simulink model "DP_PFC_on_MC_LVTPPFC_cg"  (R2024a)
settings: Solver=FixedStepDiscrete  StartTime=0.0  StopTime=0.2  FixedStep=10e-6  RelTol=1e-3  EnableMultiTasking=on
model workspace (MAT data in the model file):
  Freq = 100
  Phas = 0
  SinFreq_1 = 250
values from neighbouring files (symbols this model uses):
  ADC = ADCType.Noise    [TotemPole_PFCData.m]
  Control = ControlType.Simple    [TotemPole_PFCData.m]
  Tsc_slow = 0.01    [TotemPole_PFCData.m]
undefined symbols (not defined in the file or in its folder): a, A0, A8, AD1, AD2, AD3, AD4, AD5, address, also, AN11, AN2, AN3, AN5, AN6, AppData, as, B0, B10, B11, B7, B8, below, bin2dec, bit, bits, BOR, C, C6, C7, C9, cause, characters, Code, Communicate, contains, counter, D, D4, Data, data, dead, default, Detailed, deviced, disasserted, DS70005539, dsPIC33AK128MC106, EC, ECIO, ensure, events, Family, faster, Floating, fulll, highest, HS, HS3, I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
libraries: MCHP_Blockset x16, simulink x4, dspswit3 x1
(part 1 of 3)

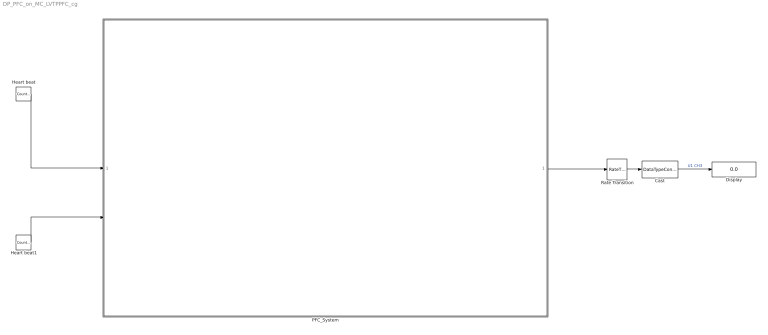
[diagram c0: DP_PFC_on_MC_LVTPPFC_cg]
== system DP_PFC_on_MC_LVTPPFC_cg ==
  Cast : DataTypeConversion  OutDataTypeStr=single
  Display : Display
  Heart beat : simulink/Sources/Counter Free-Running  NumBits=1  tsamp=.25
  Heart beat1 : simulink/Sources/Counter Free-Running  NumBits=1  tsamp=.125
  PFC_System : Subsystem
  Rate Transition : RateTransition  OutPortSampleTime=1
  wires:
  Heart beat/1 -> PFC_System/1(LED2 PIM)
  Heart beat1/1 -> PFC_System/2(LED0 Board)
  PFC_System/1(MCU load) -> Rate Transition/1
  Cast/1 -> Display/1  "U1 CH3"
  Rate Transition/1 -> Cast/1

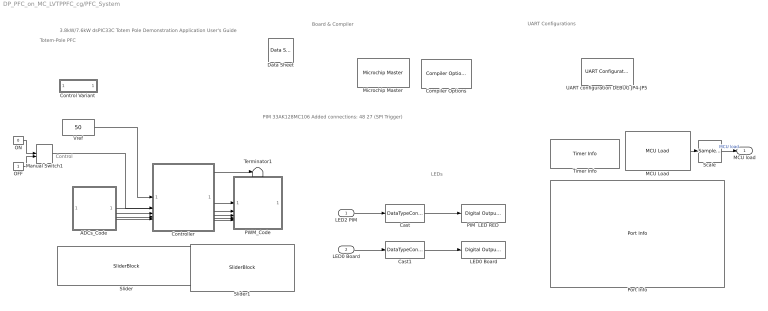
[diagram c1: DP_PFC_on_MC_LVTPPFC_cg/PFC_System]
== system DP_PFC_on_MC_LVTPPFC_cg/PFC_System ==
  note: 3.8kW/7.6kW dsPIC33C Totem Pole Demonstration Application User's Guide
  note: PIM 33AK128MC106 Added connections: 48 27 (SPI Trigger)
  note: UART Configurations
  note: LEDs
  note: Board & Compiler
  note: Control
  note: Totem-Pole PFC
  LED2 PIM : Inport
  LED0 Board : Inport  Port=2
  " LED0 Board" : MCHP_Blockset/Digital IO/Digital Output Write  PORT=Dynamic Options  PORT_TXT="C   [ 0 : 11 ]"  PIN=11  INIT_VALUE=-1  PACK=off  OUTPUT_PIN_MODE=Push-Pull (default)  SIMULTANEOUS=off  ORDERING=None  SampleTime=-1  MCHP_PORT={Digital Out}{DOU}1:1:C11;  MCHP_MASTERLINK=TotemPole_PFC_CodeGen/PFC_System/Control Variant /Microchip Master1
  ADCs_Code : Subsystem  VariantControl=ADC == 3
  Cast : DataTypeConversion  OutDataTypeStr=boolean
  Cast1 : DataTypeConversion  OutDataTypeStr=boolean
  Compiler Options : MCHP_Blockset/System Configuration/Compiler Options  Priority=1  LATEST_CMPLR=off  COMP_LIST=Dynamic Options  COMP_LIST_TXT=XC-DSC - v3.19  DFP_LIST=Dynamic Options  DFP_LIST_TXT=v 1.0.33  CMSIS_DSP=Dynamic Options  CMSIS_DSP_TXT=Dynamic Options  USE_64BIT_DOUBLE=on  MCHP_MULTITHREAD_COMPILATION=on  UseCustom_LinkerScript=off  MCHP_MASTERLINK=TotemPole_PFC_CodeGen/PFC_System/Control Variant /Microchip Master1  OPTIMIZATION_LEVEL=3  MPLAB_LINKLIB=default  MPLAB_LINKLIB1=default  CodeReplacement=Dynamic Options  CodeReplacement_TXT=None  OPTIMIZATION_FLTO=on  OPTIMIZATION_REORDER=off  OPTIMIZATION_ASM_REORDER=on  UNROLL_LOOPS=off  PROCEDURAL_ABSTRACTION=off  CONSERVE_STACK=off  GC_SECTIONS=None  MCODE=is less than 32768 (faster)  MCONST=in code memory  MDATA=Can use all available memory  MSCALAR=Use only memory below address 8192 (faster)  MLARGEARRAY=off  MAGGREGATE=on  HEAP_SIZE=0  OMF=elf  DEBUG_INFO=on  MCHP_STACK_USAGE=off  GCC_STACK_USAGE=off  ProduceHexOutput=off  AssemblyListing=off  SaveTemps=off  NO_EDS_WARN=on  PRINT_STATISTICS=off
  "Control Variant " : Subsystem  mask(Variant Selections){ControlVar=Detailed, IControlVar=PI}
      mask prompts: ControlVar "Control Variant"; IControlVar "IControl Variant"
      mask help: Select the configuration variants here.
  Controller : Subsystem  TreatAsAtomicUnit=on  ReferencedSubsystem=Control
  Data Sheet : MCHP_Blockset/System Info/Data Sheet  DOC_Type=datasheet  DOC_MCHP_Id=33AK128MC106_datasheet  DOC_FilePath=C:\Users\m67135\AppData\Local\Temp\dsPIC33AK128MC106-Family-Data-Sheet-DS70005539.pdf  DOC_FileLastCheckTime="[2024             11             14             11             58         37.374]"  cpy_MCHP_Id=33AK128MC106  MCHP_MASTERLINK=TotemPole_PFC_CodeGen/PFC_System/Control Variant /Microchip Master1
  MCU Load : MCHP_Blockset/Profiling/MCU Load  MCULoadPin=Dynamic Options  MCULoadPin_TXT=None  MCULoadMeasure=on  TIMER_Resolution=Dynamic Options  TIMER_Resolution_TXT="Resol: 0.005(us)  -  Max: 0.328(ms)"  MCHP_TIMER_REQUEST={MCU_Load}{MCU_Load}21:5:0:0:[]:32768;  MCHP_TIMER_RESULT=[2 65535 ]  MCHP_MASTERLINK=TotemPole_PFC_CodeGen/PFC_System/Control Variant /Microchip Master1  MCHP_COMPILED_INFO="CompiledSampleTime= [0.00020000000000000000958   0 ];CompiledInportDataTypes=[    ];CompiledInportDataWidth=[];"  Info="Timer 2:  Resol: 5(ns)  -  Max: 327.68(us)"  SampleTime=.0002
  Manual Switch1 : ManualSwitch  CurrentSetting=0
  Microchip Master : MCHP_Blockset/System Configuration/Microchip Master  Priority=1  PICREF=33AK128MC106  TIMESTEP_REF=PWM1_Trg1 + ADC  BUSYFLAG=Dynamic Options  BUSYFLAG_TXT=B10 / Pin[31]  VDD_range=Dynamic Options  PWRTEN=Not used  BOREN=Disable  BODENV=2.7V  BORV=Not used  FPWRT=128ms  DSBOREN=Enable ZPBOR during Deep Sleep Mode  DSLPBOR=Not used  MCLRE=Enabled  SMCLR=MCLR pin generates a normal system Reset  PMDL1WAY=Allow only one reconfiguration  RSTPRI=Device will obtain reset instruction from Primary flash  TEMP=Not used  SOSCSRC=Not used  SOSCSEL=Not used  IOL1WAY=Allow only one reconfiguration  ALTVREF=Not used  DISUVREG=Not used  DSSWEN=Not used  LPCFG=Not used  RTCBAT=Not used  VBTBOR=Not used  WUTSEL=Not used  POWERSAVE=off  FNOSC=Primary Oscillator (XT; HS; EC)  FPR=ECIO w/ PLL 16x  FOSFPR=HS3 w/PLL 16x  FOS=Primary Oscillator  FRANGE=High Range  OSCILLATOR_SELECT=External Clock  OSCILLATOR_SELECT_spd=External Clock  QUARTZ=8e6  QUARTZ_spd=8e6  POSCGAIN=2x gain setting  POSCBOOST=Boost the kick start of the oscillator  SOSCGAIN=2x gain setting  SOSCBOOST=Boost the kick start of the oscillator  ACTIV_PLL=on  ACTIV_PLL_spd=on  MIPS_DESIRED=200e6  MIPS_DESIRED_spd=200e6  CPUDIV=Divide by 1  FPLLMUL=Not used  FPLLIDIV=8x Divider  POSCFREQ=Not used  POSCMD=EC (External Clock) Mode  POSCMOD=Primary Oscillator Disabled  MIPS=200 * 1e6  ACLKCON=Optimized for PWM resolution & ADC conversion speed  ACLKCON_spd=Optimized for PWM resolution & ADC conversion speed  FPLLODIV=32x Divider  PLLKEN=PLL lock signal will be used to disable PLL clock output if lock is lost  FCKSM=Both Clock switching and Fail-safe Clock Monitor are enabled  FCKSMEN=Sw Disabled; Mon Disabled  IESO=Start up with FRC; then switch  DSWDTPS=1:2^36  FWDTEN=WDT controlled via SW; use WDTCON.ON bit  FWDTWINSZ=Window size is 25%  FWPSA=1:512  FWPSA0=1:128  FWPSB=1:16  WDT=Disable  WDTPOST=1:32768  WDTPRE=1:128  WDTPS=1:32768  WINDIS=Watchdog Timer operates in Non-Window mode  WWDTEN=Non-Window mode  DSWDTEN=Enable DSWDT during Deep Sleep Mode  DSWDTOSC=Select LPRC as DSWDT Reference clock  FWDT_RCLKSEL=WDT Run Mode uses BFRC:256  FWDT_RWDTPS=1:2147483648  FWDT_SWDTMPS=1:2147483648  FWDT_WDTEN=WDT is controlled by software; use WDTCON.ON bit  FWDT_WDTRSTEN=WDT event generates a reset  FWDT_WDTWIN=WDT Window is 25% of WDT period  FWDT_WINEN=Watchdog Timer operates in Window mode  FPBDIV=Not used  FSOSCEN=Disable Secondary Oscillator  LPRCSEL=Not used  OSCIOFCN=Not used  OSCIOFNC=general purpose digital I/O pin  LVRCFG=Not used  PLL_96MHZ=Not used  PLL96MHZ=Not used  PLLDIV=Not used  WDTCLK=Not used  WDTCMX=Not used  WDTWIN=WDT Window is 25% of WDT period  XTCFG=24-32 MHz crystals  XTBST=Boost the kick-start  APL=Aux Flash Code protect is disabled  APLK=Aux Flash Write Protection or Code Protection is Enabled  AWRP=Auxiliary program memory is not write-protected  BSS=No Protection (other than BWRP)  BWP=Not used  BWRP=Boot Segment may be written  CP=Protection Disabled  EBS=No Boot EEPROM  ESS=No Segment Data EEPROM  GCP=General Segment Code protect is Disabled  GSS=No Protection (other than GWRP)  GSS0=Not used  GSSK=General Segment Write Protection or Code Protection is Enabled  GWRP=General Segment may be written  PWP=Not used  RBS=No Boot RAM  RSS=No Secure RAM  SSS=No Secure Segment  SWRP=Secure segment may be written  WPCFG=Not used  WPDIS=Not used  WPEND=Not used  WPFP=Not used  ICESEL=Communicate on PGEC1/PGED1  ICS=Communicate on PGC2 and PGD2  JTAGEN=Disable  FICD_JTAGEN=Disable  COE=Not used  RES=Not used  DEBUG=Debugger is disabled  BACKBUG=Not used  BKBUG=Not used  ALTI2C=I2C mapped to SDA1/SCL1 pins  ALTI2C1=I2C1 mapped to SDA1/SCL1 pins  ALTI2C2=I2C2 mapped to SDA2/SCL2 pins  ALTI2C3=I2C3 mapped to SDA3/SCL3 pins  FDEVOPT1_ALTI2C1=Not used  FDEVOPT1_ALTI2C2=Not used  FDEVOPT1_SPI2MAPDIS=Not used  FDEVOPT_ALTI2C1=Primary I2C1 pins are used  FDEVOPT_ALTI2C2=Primary I2C2 pins are used  FDEVOPT_ALTI2C3=Primary I2C3 pins are used  FDEVOPT_SPI2PIN=SPI2 pins are selected by peripheral pin selection feature  ALTQIO=QEA1; QEB1; INDX1 are selected as inputs to QEI1  ALTSS1=SS1A is selected as the I/O pin for SPI1  CMPPOL0=Hysteresis is applied to falling edge  CMPPOL1=Hysteresis is applied to falling edge  FCANIO=Not used  FETHIO=Default Ethernet I/O  FMIIEN=MII Enabled  FSRSSEL=Not used  FUSBIDIO=Controlled by the USB Module  FVBUSONIO=Not used  HPOL=PWM module high side output pins have active-high output polarity  HYST0=45 mV Hysteresis  HYST1=45 mV Hysteresis  I2C1SEL=Not used  LPOL=PWM module low side output pins have active-high output polarity  PWMPIN=PWM module pins controlled by PORT register at device Reset  RTCOSC=Not used  UPLLEN=USB PLL Disabled  UPLLIDIV=Not used  ATMOD8=Not used  ALTPMP=Not used  I2C2SEL=Not used  ALTADREF=Not used  ALTCVREF=Not used  PWMLOCK=PWM registers may be written without key sequence  INT_PRIORITY_DMA=0  MCHP_TIMER_RESULT=[ ]  MCHP_PORT={Busy Flag}{Busy}0:1:B10;  MCHP_PLLRegisters="[0        -1     16386        -1  16815713]"  MCHPVAR=MCHP.fcy.MIPS=2e+08;MCHP.fcy.SYSCLK=2e+08;MCHP.fcy.Fplli=8000000;MCHP.fcy.Fvco=1.2e+09;MCHP.fcy.Fpllo=2e+08;MCHP.fcy.PWM=2e+08;MCHP.fcy.ADC=80000000;MCHP.fcy.UART=2e+08;MCHP.fcy.SPI=2e+08;MCHP.fcy.SCC=2e+08;MCHP.fcy.Timers=1e+08;MCHP.fcy.I2C=2e+08;MCHP.PowerSave=0;MCHP.TimeStepFactor=MCHP_Fun.Hex2num('C0F869FFFFFFFFFF');MCHP.TimeStep_Timer=-1;MCHP.NTIMERS=1;MCHP.id.name='33AK128MC106';MCHP.id.N=re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  MCHP_CRC=19172077  BTMODE=Device is in Single Boot (legacy) mode  RES1=Not used  PLLSS=Not used  RES2=Not used  ALTCMPI=Not used  BOREN1=Not used  ALTRB6=Not used  RETCFG=Not used  DFMCY=Not used  BSS2=No Boot Segment  BSEN=No Boot Segment  CWRP=Configuration Segment may be written  CSS=No Protection (other than CWRP)  AIVTDIS=Disabled AIVT  BSLIM=Not used  WDTEN=Disable  BTSWP=BOOTSWP instruction is disabled  DBCC=No Cross Connection between DAC outputs  CTXT1=Not Assigned  CTXT2=Not Assigned  SEQNUM=Not used  nSEQNUM=Not used  BOREN0=Enabled  DMTIVT=Not used  DMTCNT=2^31 (2147483648)  DMTEN=Dead Man Timer is Disabled and can be enabled by software  ON=Not used  USERID=Not used  RESERVED1=Not used  PGL1WAY=Allow only one reconfiguration  FPLLRNG=34-68 MHz Input  FPLLICLK=FRC is input to the System PLL  FPLLMULT=PLL Multiply by 128  UPLLFSEL=USB PLL input is 24 MHz  DMTINTV=Window/Interval value is 127/128 counter value  WDTSPGM=WDT stops during Flash programming  FDMTEN=Deadman Timer is disabled  TRCEN=Trace features in the CPU are enabled  BOOTISA=Boot code and Exception code is MIPS32  FECCCON=ECC and Dynamic ECC are disabled (ECCCON bits are writable)  EXTDDRSIZE=Not used  FSLEEP=Flash is powered down when the device is in Sleep mode  DBGPER=Allow CPU access to all permission regions  EJTAGBEN=Normal EJTAG functionality  TSEQ=Not used  CSEQ=Not used  RWDTPS=1:1048576  RCLKSEL=Always use LPRC  SWDTPS=1:1048576  DMTIVTL=Not used  DMTIVTH=Not used  DMTCNTL=Not used  DMTCNTH=Not used  DMTDIS=Dead Man Timer is Disabled and can be enabled by software  SMBEN=SMBus input threshold is enabled  SPI2PIN=SPI2 uses I/O remap (PPS) pins  CTXT3=Not Assigned  CTXT4=Not Assigned  MBXM0=Mailbox register configured for Main data read (Secondary to Main data transfer)  MBXM1=Mailbox register configured for Main data read (Secondary to Main data transfer)  MBXM2=Mailbox register configured for Main data read (Secondary to Main data transfer)  MBXM3=Mailbox register configured for Main data read (Secondary to Main data transfer)  MBXM4=Mailbox register configured for Main data read (Secondary to Main data transfer)  MBXM5=Mailbox register configured for Main data read (Secondary to Main data transfer)  MBXM6=Mailbox register configured for Main data read (Secondary to Main data transfer)  MBXM7=Mailbox register configured for Main data read (Secondary to Main data transfer)  MBXM8=Mailbox register configured for Main data read (Secondary to Main data transfer)  MBXM9=Mailbox register configured for Main data read (Secondary to Main data transfer)  MBXM10=Mailbox register configured for Main data read (Secondary to Main data transfer)  MBXM11=Mailbox register configured for Main data read (Secondary to Main data transfer)  MBXM12=Mailbox register configured for Main data read (Secondary to Main data transfer)  MBXM13=Mailbox register configured for Main data read (Secondary to Main data transfer)  MBXM14=Mailbox register configured for Main data read (Secondary to Main data transfer)  MBXM15=Mailbox register configured for Main data read (Secondary to Main data transfer)  MBXHSA=MSIxMBXD15 assigned to mailbox handshake protocol block A  MBXHSB=MSIxMBXD15 assigned to mailbox handshake protocol block B  MBXHSC=MSIxMBXD15 assigned to mailbox handshake protocol block C  MBXHSD=MSIxMBXD15 assigned to mailbox handshake protocol block D  MBXHSE=MSIxMBXD15 assigned to mailbox handshake protocol block E  MBXHSF=MSIxMBXD15 assigned to mailbox handshake protocol block F  MBXHSG=MSIxMBXD15 assigned to mailbox handshake protocol block G  MBXHSH=MSIxMBXD15 assigned to mailbox handshake protocol block H  HSAEN=Mailbox data flow control handshake protocol block disabled  HSBEN=Mailbox data flow control handshake protocol block disabled  HSCEN=Mailbox data flow control handshake protocol block disabled  HSDEN=Mailbox data flow control handshake protocol block disabled  HSEEN=Mailbox data flow control handshake protocol block disabled  HSFEN=Mailbox data flow control handshake protocol block disabled  HSGEN=Mailbox data flow control handshake protocol block disabled  HSHEN=Mailbox data flow control handshake protocol block disabled  CPRA0=Main core owns pin  CPRA1=Main core owns pin  CPRA2=Main core owns pin  CPRA3=Main core owns pin  CPRA4=Main core owns pin  CPRB0=Main core owns pin  CPRB1=Main core owns pin  CPRB2=Main core owns pin  CPRB3=Main core owns pin  CPRB4=Main core owns pin  CPRB5=Main core owns pin  CPRB6=Main core owns pin  CPRB7=Main core owns pin  CPRB8=Main core owns pin  CPRB9=Main core owns pin  CPRB10=Main core owns pin  CPRB11=Main core owns pin  CPRB12=Main core owns pin  CPRB13=Main core owns pin  CPRB14=Main core owns pin  CPRB15=Main core owns pin  CPRC0=Main core owns pin  CPRC1=Main core owns pin  CPRC2=Main core owns pin  CPRC3=Main core owns pin  CPRC4=Main core owns pin  CPRC5=Main core owns pin  CPRC6=Main core owns pin  CPRC7=Main core owns pin  CPRC8=Main core owns pin  CPRC9=Main core owns pin  CPRC10=Main core owns pin  CPRC11=Main core owns pin  CPRC12=Main core owns pin  CPRC13=Main core owns pin  CPRC14=Main core owns pin  CPRC15=Main core owns pin  CPRD0=Main core owns pin  CPRD1=Main core owns pin  CPRD2=Main core owns pin  CPRD3=Main core owns pin  CPRD4=Main core owns pin  CPRD5=Main core owns pin  CPRD6=Main core owns pin  CPRD7=Main core owns pin  CPRD8=Main core owns pin  CPRD9=Main core owns pin  CPRD10=Main core owns pin  CPRD11=Main core owns pin  CPRD12=Main core owns pin  CPRD13=Main core owns pin  CPRD14=Main core owns pin  CPRD15=Main core owns pin  CPRE0=Main core owns pin  CPRE1=Main core owns pin  CPRE2=Main core owns pin  CPRE3=Main core owns pin  CPRE4=Main core owns pin  CPRE5=Main core owns pin  CPRE6=Main core owns pin  CPRE7=Main core owns pin  CPRE8=Main core owns pin  CPRE9=Main core owns pin  CPRE10=Main core owns pin  CPRE11=Main core owns pin  CPRE12=Main core owns pin  CPRE13=Main core owns pin  CPRE14=Main core owns pin  CPRE15=Main core owns pin  S1FNOSC=Internal Fast RC (FRC) Oscillator with postscaler  S1IESO=Start up with FRC; then switch  S1OSCIOFNC=OSC2 is clock output  S1FCKSM=Both Clock switching and Fail-safe Clock Monitor are disabled  S1PLLKEN=S1PLLKEN_ON  S1RWDTPS=1:1048576  S1RCLKSEL=Always use LPRC  S1WINDIS=Watchdog Timer operates in Non-Window mode  S1WDTWIN=WDT Window is 25% of WDT period  S1SWDTPS=1:1048576  S1FWDTEN=use WDTCON.ON bit  S1ICS=Communicate on PGC3 and PGD3  S1DEBUG=Not used  S1ISOLAT=The Secondary can operate (in debug mode) even if the SLVEN bit in the MSI is zero  S1NOBTSWP=BOOTSWP instruction is disabled  S1ALTI2C1=I2C1 mapped to SDA1/SCL1 pins  S1SPI1PIN=Secondary SPI1 uses I/O remap (PPS) pins  S1SSRE=Secondary generated resets will reset the Secondary Enable Bit in the MSI module  S1MSRE=The Main software oriented RESET events (RESET Op-Code; Watchdog timeout; TRAP reset; illegalInstruction) will also cause the Secondary subsystem to reset  S1CTXT1=Not Assigned  S1CTXT2=Not Assigned  S1CTXT3=Not Assigned  S1CTXT4=Not Assigned  BORLVL=Not used  BSSO=Not used  MCA=Not used  MAXTEMP=Not used  CFGAN14=Not used  CFGAN15=Not used  S1IOL1WAY=Not used  S1BSSO=Not used  S1BACKBUG=Not used  BISTDIS=mBIST on reset feature disabled  NOBTSWP=BOOTSWP instruction is disabled  S1BISTDIS=Secondary BIST on reset feature disabled  S1DMTIVTL=Not used  S1DMTIVTH=Not used  S1DMTCNTL=Not used  S1DMTCNTH=Not used  S1DMTDIS=Secondary Dead Man Timer is Disabled and can be enabled by software  BSEQ=Not used  IBSEQ=Not used  SMB3EN=SMBus 3.0 input levels  FUSBIDIO2=USBID pin is controlled by the USB2 module  FVBUSIO2=VBUSON pin is controlled by the USB2 module  FUSBIDIO1=USBID pin is controlled by the USB1 module  FVBUSIO1=VBUSON pin is controlled by the USB1 module  VBATBOREN=Enable ZPBOR during VBAT Mode  FDSEN=Enable DSEN bit in DSCON  BORSEL=BOR trip voltage 2.1v (Non-OPAMP deviced operation)  POSCFGAIN=Gain is G3  POSCAGCDLY=Settling time = 25ms x AGCRNG  POSCAGCRNG=Range 1x  POSCAGC=Automatic Gain Control for Oscillator  FDBGWP=Not used
  OFF : Constant  OutDataTypeStr=single  SampleTime=Tsc_slow
  ON : Constant  Value=0  OutDataTypeStr=single  SampleTime=Tsc_slow
  PIM  LED RED : MCHP_Blockset/Digital IO/Digital Output Write  PORT=Dynamic Options  PORT_TXT="D   [ 0 : 12 ]"  PIN=11  INIT_VALUE=-1  PACK=off  OUTPUT_PIN_MODE=Push-Pull (default)  SIMULTANEOUS=off  ORDERING=None  SampleTime=-1  MCHP_PORT={Digital Out}{DOU}1:1:D11;  MCHP_MASTERLINK=TotemPole_PFC_CodeGen/PFC_System/Control Variant /Microchip Master1
  PWM_Code : Subsystem  VariantControl=PWM == 3  mask(PWM Generator for Totem Pole PFC Converter){}
  Port Info : MCHP_Blockset/System Info/Port Info  MCHP_MASTERLINK=TotemPole_PFC_CodeGen/PFC_System/Control Variant /Microchip Master1
  Scale : SampleTimeMath  TsampMathOp=/  weightValue=inv(5e-9)  OutDataTypeStr=fixdt(0,16,15)  RndMeth=Round  SaturateOnIntegerOverflow=on
  Slider : SliderBlock  ScaleMin=50  ScaleMax=60
  Slider1 : SliderBlock  ScaleMin=5  ScaleMax=15
  Terminator1 : Terminator
  Timer Info : MCHP_Blockset/System Info/Timer Info  MCHP_MASTERLINK=TotemPole_PFC_CodeGen/PFC_System/Control Variant /Microchip Master1
  UART configuration DEBUG JP4-JP5 : MCHP_Blockset/BUS UART/UART Configuration  UART_REF=1  BAUD_Choice=Dynamic Options  BAUD_Choice_TXT="460800         [+0.01%]"  BAUD_Choice_IR=Dynamic Options  BAUD_Choice_IR_TXT=[]  BAUD_Custom=115200  INT_PRIORITY=0  ALT_IO=on  PIN_RX=Dynamic Options  PIN_RX_TXT=C6 / P39 / Pin[35]  PIN_RX_INPUT_MODE=Hi-impedance (default)  PIN_TX=Dynamic Options  PIN_TX_TXT=C7 / P40 / Pin[36]  PIN_TX_OUTPUT_MODE=Push-Pull (default)  MCHP_PORT="{UART1  Rx}{U1RX}3:0:P39;{UART1  Tx}{U1TX}3:0:P40;"  MCHP_MASTERLINK=TotemPole_PFC_CodeGen/PFC_System/Control Variant /Microchip Master1  MCHP_COM_ExtPil=on  TX_IMPLEMENTATION=Circular Buffer  TX_IMPLEMENTATION_default=Circular Buffer  TX_INT_PRIORITY=5  TX_INT_WHEN=is empty & last char is sent  TX_INT_WHEN_default=is empty & last char is sent  TX_CIRCULAR_SIZE=256  TX_DMA_CHANNEL="0   (Lowest Priority)"  TX_DMA_SIZE=512  TX_TASK_PROTECTION=Delay tasks (default)  TX_INTERRUPT_PROTECTION=Do not send on conflict (default)  TX_INTERRUPT_PROTECTION_default=Do not send on conflict (default)  RX_IMPLEMENTATION=Circular Buffer  RX_IMPLEMENTATION_default=Circular Buffer  RX_INT_PRIORITY=5  RX_INT_WHEN=is 3/4 fulll (contains 3 data characters)  RX_CIRCULAR_SIZE=64  RX_DMA_CHANNEL=0  RX_DMA_SIZE=0  DuplexMode=Full duplex (default)  PIN_RX_Inv=off  PIN_TX_Inv=off  PIN_RXTX_Inv=off  ParityBit=No parity (default)  StopBit=1 stop bit (default)  IRDA=off  IdleTime_choice=Dynamic Options  IdleTime_choice_TXT=None  IdleTime_custom=2/50  FlowControl=None  PIN_CTS=Dynamic Options  PIN_CTS_TXT=B0 / P17 / Pin[20]  PIN_CTS_INPUT_MODE=Hi-impedance (default)  PIN_RTS=Dynamic Options  PIN_RTS_TXT=B0 / P17 / Pin[20]  PIN_RTS_OUTPUT_MODE=Push-Pull (default)  PIN_DSR=Dynamic Options  PIN_DSR_TXT=B0 / P17 / Pin[20]  PIN_DSR_INPUT_MODE=Hi-impedance (default)  PIN_DTR=Dynamic Options  PIN_DTR_TXT=B0 / P17 / Pin[20]  PIN_DTR_OUTPUT_MODE=Push-Pull (default)  InitSequence_chkbox=off  BAUD_Choice_InitSeq=Dynamic Options  BAUD_Choice_InitSeq_TXT="115200         [+0.01%]"  BAUD_Choice_IR_InitSeq=Dynamic Options  BAUD_Choice_IR_InitSeq_TXT=0  BAUD_Custom_InitSeq=0  InitSequence="uint8(['use VT100 terminal ! ' 13 10 27 'c'  27 '[2J' ] )"
  Vref : Constant  Value=50  OutDataTypeStr=single  SampleTime=Tsc_slow
  MCU load : Outport
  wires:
  MCU Load/1 -> Scale/1
  Scale/1 -> MCU load/1  "MCU load"
  LED0 Board/1 -> Cast1/1
  LED2 PIM/1 -> Cast/1
  Cast/1 -> PIM  LED RED/1
  Cast1/1 -> " LED0 Board"/1
  OFF/1 -> Manual Switch1/2
  ON/1 -> Manual Switch1/1
  Vref/1 -> Controller/1
  ADCs_Code/1("Vin ") -> Controller/3
  Manual Switch1/1 -> Controller/2
  ADCs_Code/2("Vout ") -> Controller/4
  ADCs_Code/3("Iac ") -> Controller/5
  Controller/7 -> ADCs_Code/1(I_est_offset)
  Controller/1 -> Terminator1/1
  Controller/2 -> PWM_Code/1(DC)
  Controller/3 -> PWM_Code/2(v_pos1)
  Controller/4 -> PWM_Code/3(v_neg2)
  Controller/5 -> PWM_Code/4(v_zc1)
  Controller/6 -> PWM_Code/5(PWM_Mode)
